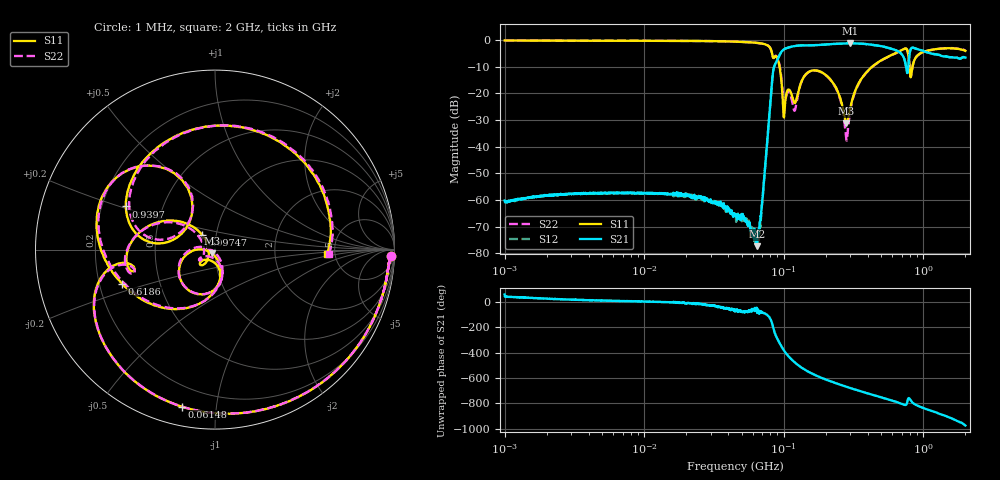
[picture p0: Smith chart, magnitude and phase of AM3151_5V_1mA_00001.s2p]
! Date/Time: Fri Jun 26 10:21:57 2020
! Network Analyzer:  Rev:
! Sweep from 1000000.0 to 2000000000.0, 1601 Points ! Power Supply: 0 V, 0 A
# HZ S DB R 50
!freq MagS11 AngS11 MagS21 AngS21 MagS12 AngS12 MagS22 AngS22
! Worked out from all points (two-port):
!   1601 points, 1 MHz to 2 GHz, reference 50 ohm
!   highest |S21| = -1.24 dB at 297.7 MHz (marker M1); lowest = -77.3 dB at 64.47 MHz (marker M2)
!   |S21| within 3 dB of the highest: 96.83 MHz to 660.1 MHz (563.3 MHz wide, 149 % of centre); 802.9 MHz to 1.014 GHz (211.4 MHz wide, 23.3 % of centre)
!   lowest |S11| = -31.2 dB at 281.2 MHz (marker M3), VSWR 1.06, Z = 48.2 - j2.01 ohm
!   |S11| at or under -10 dB: 93.27 MHz to 430 MHz (336.8 MHz wide, 129 % of centre); 795.9 MHz to 836 MHz (40.07 MHz wide, 4.91 % of centre)
!   |S22| runs from -37.7 to -0.2 dB; largest |S21 - S12| = 0.01
!   S11 on the Smith chart (normalised r, x): 1 MHz: 23, -42; 61.48 MHz: 0.09, -0.81; 97.47 MHz: 0.85, +0.14; 618.6 MHz: 0.30, -0.16; 939.7 MHz: 0.30, +0.21; 2 GHz: 4.32, -0.32
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1000000  -0.18 -2.1  -60.22 55.8  -60.53 38.0  -0.17 -2.1
3555161  -0.26 -5.7  -57.52 13.9  -57.56 12.9  -0.25 -5.7
1.263916e7  -0.30 -19.2  -57.45 -2.4  -57.47 -1.2  -0.30 -19.1
4.493426e7  -0.59 -70.3  -65.73 -63.1  -65.94 -67.8  -0.61 -70.3
6.148155e7  -0.98 -101.9  -74.98 -59.7  -76.34 -62.1  -0.98 -102.0
6.447278e7  -1.09 -108.7  -77.30 -89.3  -76.40 -104.3  -1.08 -108.6
6.890648e7  -1.28 -119.8  -64.19 -75.8  -65.42 -84.9  -1.29 -119.7
8.372392e7  -6.51 -169.7  -12.15 162.1  -12.14 162.1  -6.50 -168.5
9.03357e7  -7.10 169.1  -7.18 63.2  -7.18 63.2  -6.85 171.5
9.746975e7  -19.17 131.1  -4.05 -1.9  -4.06 -2.0  -17.31 139.6
1.156494e8  -21.70 -135.4  -2.41 -102.2  -2.41 -102.2  -23.85 -145.0
1.589914e8  -11.47 -112.6  -1.98 155.0  -1.97 154.9  -11.51 -113.1
2.313992e8  -17.00 -173.9  -1.46 82.3  -1.46 82.3  -17.22 -179.5
2.811581e8  -31.24 -130.6  -1.28 50.8  -1.26 51.0  -37.62 -134.3
2.976517e8  -26.06 -79.7  -1.24 42.1  -1.24 42.0  -27.31 -64.2
3.633796e8  -14.21 -84.8  -1.42 12.3  -1.43 12.4  -14.32 -82.3
5.652395e8  -6.13 -145.9  -2.99 -49.9  -2.97 -49.8  -6.19 -147.2
6.186321e8  -5.18 -159.9  -3.62 -62.7  -3.61 -62.7  -5.24 -161.6
7.624488e8  -3.49 140.3  -12.00 -77.5  -12.00 -77.4  -3.66 137.2
9.397004e8  -5.16 154.2  -3.66 -104.4  -3.69 -104.5  -5.21 150.6
1.400532e9  -3.16 80.5  -6.13 -172.8  -6.12 -173.0  -3.10 77.2
2e9  -4.07 -2.1  -6.60 107.0  -6.72 106.6  -3.91 -2.3
